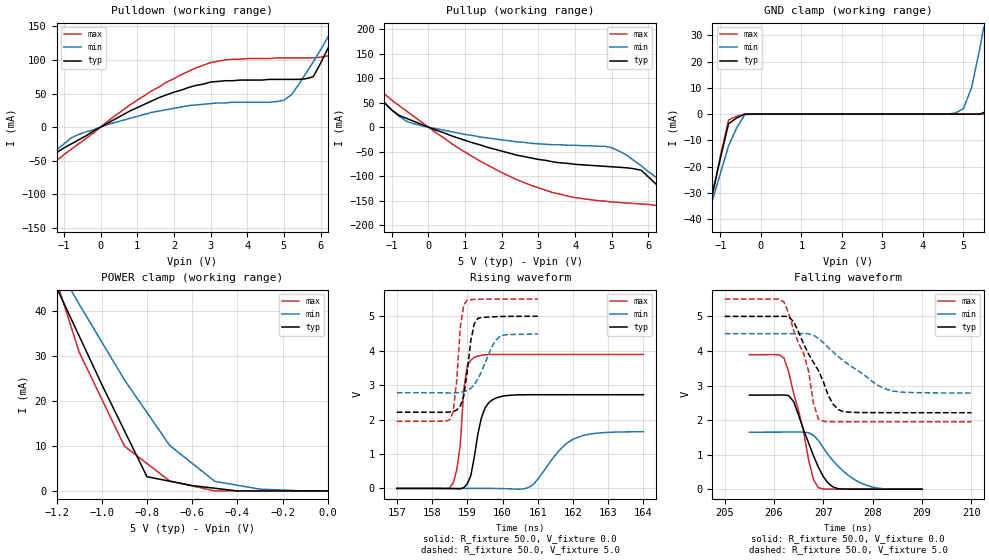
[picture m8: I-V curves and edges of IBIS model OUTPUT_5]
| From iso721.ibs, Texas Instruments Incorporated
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|   Output 5.0V
[Model]   OUTPUT_5
Model_type   3-state
Vmeas = 2.2V   |Reference voltage for timing measurements
Cref = 15pF   |Timing specification test load capacitance value
Vref = 0   |Timing specification test load voltage; GND
| variable   typ   min   max
C_comp   2.1pF   1.7pF   2.5pF
|   typ   min   max
[Temperature Range]   25.0   -40   125
[Voltage range]   5.0V   4.5V   5.5V
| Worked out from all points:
|   slope of the pulldown table from 0 to 0.75 V, typ, clamps not added: 33.3 ohm
|   slope of the pullup table from 0 to 0.75 V, typ, clamps not added: 36.1 ohm
|   GND clamp passes 1 mA (typ) near -0.54 V on its own axis
|   POWER clamp passes 1 mA (typ) near -0.57 V on its own axis
|   rising waveform, R_fixture 50.0, V_fixture 0.0: 20-80 % time 315ps typ, 793ps min, 200ps max; typ from 0 V to 2.72 V
|   falling waveform, R_fixture 50.0, V_fixture 0.0: 20-80 % time 444ps typ, 634ps min, 370ps max; typ from 2.72 V to 0 V
|   rising waveform, R_fixture 50.0, V_fixture 5.0: 20-80 % time 219ps typ, 451ps min, 171ps max; typ from 2.21 V to 5 V
|   falling waveform, R_fixture 50.0, V_fixture 5.0: 20-80 % time 556ps typ, 928ps min, 422ps max; typ from 5 V to 2.21 V
[Pulldown]
|   Voltage   I(typ)  I(min)  I(max)
-5.5V     -360mA     -275mA     -490mA
-3.5V     -206mA     -162mA     -275mA
-2.5V     -129mA     -105mA     -169mA
-1.4V     -49mA      -45mA      -60mA
-800mV    -25mA      -16mA      -33mA
1.4V      39mA       22mA       54mA
3V        67mA       35mA       96mA
5V        71mA       40mA       103mA
5.8V      75mA       97mA       103mA
6.4V      141mA      152mA      114mA
7V        216mA      208mA      201mA
11V       766mA      612mA      949mA
[Pullup]
|   Voltage   I(typ)  I(min)  I(max)
| Note that the[Pullup]voltage table is referenced to Vcc
| and is calculated using Vtable=Vcc - Vmeasured.
-5.5V     585mA      451mA      786mA
-3V       269mA      216mA      353mA
-2.5V     207mA      170mA      267mA
-2V       144mA      123mA      182mA
-1.5V     83mA       78mA       102mA
-800mV    24mA       22mA       44mA
2.8V      -63mA      -33mA      -119mA
5V        -81mA      -42mA      -153mA
5.8V      -88mA      -79mA      -157mA
7.5V      -218mA     -177mA     -278mA
8V        -258mA     -206mA     -332mA
10.5V     -456mA     -351mA     -608mA
[GND_clamp]
|   Voltage   I(typ)   I(min)   I(max)
| Outputs in High Impedance (off)
-5.5V     -359.9mA   -275.1mA   -489.5mA
-1.4V     -44.92mA   -43.82mA   -51.83mA
-1.3V     -37.54mA   -38.38mA   -41.63mA
-1.2V     -30.16mA   -32.94mA   -31.43mA
-1V       -16.66mA   -22.42mA   -15.87mA
-800mV    -3.66mA    -12.05mA   -2.249mA
-600mV    -1.479mA   -5.279mA   -861.1uA
-400mV    -1.657uA   -187.7uA   -4.797uA
4.8V      37.53pA    388.9uA    31.79pA
5V        41.24pA    2.119mA    35.42pA
5.2V      2.711nA    10.13mA    39.28pA
5.5V      594.7uA    33.09mA    45.67pA
[POWER_clamp]
|   Voltage  I(typ)   I(min)   I(max)
| Note that the [POWER_clamp] voltage table is referenced to Vcc
| and is calculated using Vtable = Vcc - Vmeasured.
| Outputs in Tri-state.
-5.5V     585.2mA    450.6mA    785.6mA
-1.2V     45.19mA    50.27mA    46.63mA
-1.1V     34.43mA    41.5mA     30.85mA
-1V       23.66mA    33.09mA    20.41mA
-900mV    13.4mA     24.69mA    9.969mA
-800mV    3.151mA    17.41mA    6.092mA
-700mV    2.17mA     10.13mA    2.215mA
-600mV    1.189mA    6.126mA    1.108mA
-500mV    594.7uA    2.119mA    44.53nA
-400mV    8.158nA    1.254mA    22.74nA
-300mV    5.434nA    388.9uA    942.3pA
0V        41.24pA    132.3nA    45.67pA
[Ramp]
|   typ   min   max
dV/dt_r   1.63V/3.2ns   0.99V/7.9ns   2.33V/2.0ns
dV/dt_f   1.63V/4.3ns   0.99V/6.4ns   2.33V/3.7ns
R_load = 50
[Rising Waveform]
R_fixture = 50.0
V_fixture = 0.0
C_fixture = 0p
L_fixture = 0n
|   V(typ)   V(min)   V(max)
157ns     675.8pV    11.36nV    607.5pV
158.6ns   -5.929mV   23.9uV     157.7mV
158.8ns   -13.42mV   55.63uV    1.235V
159ns     130.7mV    100.2uV    3.562V
159.2ns   913.9mV    166.3uV    3.804V
159.4ns   2.047V     277.8uV    3.867V
159.8ns   2.619V     -2.05mV    3.891V
160.8ns   2.721V     61.45mV    3.893V
162.1ns   2.722V     1.469V     3.893V
164ns     2.722V     1.647V     3.893V
[Falling Waveform]
R_fixture = 50.0
V_fixture = 0.0
C_fixture = 0p
L_fixture = 0n
|   V(typ)   V(min)   V(max)
205.5ns   2.722V     1.649V     3.893V
206.2ns   2.726V     1.652V     3.8V
206.4ns   2.526V     1.654V     2.751V
206.6ns   1.714V     1.65V      1.646V
206.7ns   1.338V     1.631V     849mV
206.8ns   965.6mV    1.56V      270.5mV
206.9ns   629.7mV    1.405V     42.07mV
207.2ns   61.15mV    813.5mV    490.2uV
207.8ns   594.9uV    152.6mV    -12.38uV
209ns     -8.937uV   844.7uV    680.3nV
[Rising Waveform]
R_fixture = 50.0
V_fixture = 5.0
V_fixture_min = 4.5
V_fixture_max = 5.5
C_fixture = 0p
L_fixture = 0n
|   V(typ)   V(min)  V(max)
157ns     2.213V     2.781V     1.949V
158.5ns   2.219V     2.774V     1.991V
158.6ns   2.236V     2.775V     2.221V
158.7ns   2.278V     2.778V     3.13V
158.8ns   2.383V     2.79V      4.658V
159ns     3.417V     2.846V     5.473V
159.1ns   4.291V     2.907V     5.482V
159.3ns   4.941V     3.177V     5.494V
159.9ns   4.992V     4.395V     5.5V
161ns     5V         4.486V     5.5V
[Falling Waveform]
R_fixture = 50.0
V_fixture = 5.0
V_fixture_min = 4.5
V_fixture_max = 5.5
C_fixture = 0p
L_fixture = 0n
|   V(typ)   V(min)  V(max)
205ns     5V         4.5V       5.5V
206.2ns   5.004V     4.5V       5.419V
206.4ns   4.84V      4.501V     4.59V
206.6ns   4.202V     4.505V     3.934V
206.8ns   3.669V     4.455V     2.482V
206.9ns   3.43V      4.362V     2.029V
207.2ns   2.453V     3.964V     1.951V
207.4ns   2.245V     3.724V     1.949V
208.4ns   2.213V     2.842V     1.949V
210ns     2.213V     2.782V     1.949V
